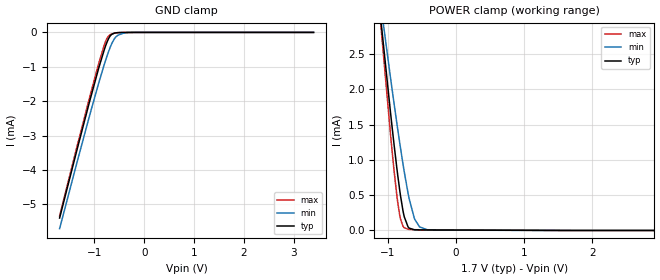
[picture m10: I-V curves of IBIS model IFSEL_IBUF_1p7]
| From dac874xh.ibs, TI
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|   IFSEL_IBUF_1p7 Model
[Model]   IFSEL_IBUF_1p7
Model_type   Input
Vinl = 0.51
Vinh = 1.19
|   typ   min   max
C_comp   1.23168E-13  1.77948E-14  2.05096E-13
| Where nom  PVT is Nominal Process, 1.7V, 27C
|   Fast PVT is Strong Process,  1.701V, -40C
|   Slow PVT is Weak Process,   1.699V, 150C
[Model spec]
|subparameter
Vinl   0.51   0.5097   0.5103
Vinh   1.19   1.1893   1.1907
[Voltage Range]   1.7   1.699   1.701
[Temperature Range]   27   150   -40
[Power Clamp Reference]   1.7   1.699   1.701
[GND Clamp Reference]   0   0   0
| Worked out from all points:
|   GND clamp passes 1 mA (typ) near -0.91 V on its own axis
|   POWER clamp passes 1 mA (typ) near -0.88 V on its own axis
[GND Clamp]
|   Voltage   I(typ)   I(min)   I(max)
-1.7V     -5.401mA   -5.709mA   -5.344mA
-1.348V   -3.401mA   -3.768mA   -3.309mA
-1.088V   -1.958mA   -2.369mA   -1.838mA
-914.6mV  -1.04mA    -1.474mA   -902.7uA
-802.4mV  -502.8uA   -931.6uA   -365.3uA
-741.2mV  -259.8uA   -660uA     -154.2uA
-685.1mV  -105.9uA   -437.9uA   -67.26uA
-603.5mV  -22.83uA   -194.3uA   -26.44uA
-532.1mV  -6.715uA   -84.04uA   -9.242uA
-419.9mV  -1.661uA   -23.09uA   -2.188uA
-256.7mV  -849.8nA   -1.349uA   -1.15uA
3.4V      0A         0A         0A
[POWER Clamp]
|   Voltage   I(typ)   I(min)   I(max)
-1.7V     8.871mA    7.745mA    9.927mA
-1.103V   2.966mA    3.18mA     2.884mA
-965.6mV  1.69mA     2.18mA     1.383mA
-909.5mV  1.202mA    1.787mA    831.1uA
-868.7mV  869.3uA    1.509mA    480.8uA
-817.7mV  498.1uA    1.174mA    166uA
-761.6mV  193.7uA    829.9uA    39.02uA
-705.5mV  49.46uA    525.1uA    17.16uA
-608.6mV  9.325uA    159.7uA    10.9uA
-537.2mV  7.601uA    50.73uA    10.13uA
-419.9mV  7.061uA    9.095uA    9.544uA
3.4V      0A         0A         0A
